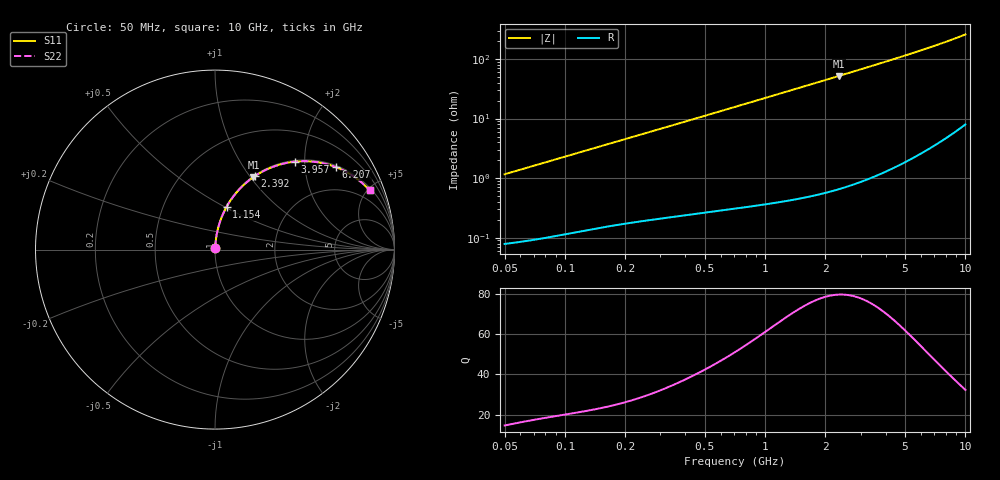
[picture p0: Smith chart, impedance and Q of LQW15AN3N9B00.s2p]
!Murata Part Number: LQW15AN3N9B00
!These Parameters are Measured in Series Mode Connection
!  o--[Z]--o
!Port1  Port2
!  o-------o
!Freq. Start=50[MHz] Stop=10[GHz], 401[Steps]
# Hz S RI R 50
!Freq.(Hz)	S 11(Real)	S 11(Imag)	S 21(Real)	S 21(Imag)	S 12(Real)	S 12(Imag)	S 22(Real)	S 22(Imag)
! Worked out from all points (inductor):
!   401 points, 50 MHz to 10 GHz, reference 50 ohm
!   read as one part in series: L = 3.68 nH near 51.34 MHz
!   highest Q = 79.5 at 2.329 GHz (marker M1), where L = 3.54 nH
!   S11 on the Smith chart (normalised r, x): 50 MHz: 1.00, +0.02; 1.154 GHz: 1.01, +0.51; 2.392 GHz: 1.01, +1.06; 3.957 GHz: 1.03, +1.78; 6.207 GHz: 1.06, +2.90; 10 GHz: 1.16, +5.16
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5e7  0.000921 0.0116  0.9991 -0.0116  0.9991 -0.0116  0.000921 0.0116
1.214486e8  0.00205 0.0276  0.9979 -0.0276  0.9979 -0.0276  0.00205 0.0276
1.956524e8  0.00364 0.0439  0.9964 -0.0439  0.9964 -0.0439  0.00364 0.0439
2.949953e8  0.00639 0.0655  0.9936 -0.0655  0.9936 -0.0655  0.00639 0.0655
4.689809e8  0.0132 0.1028  0.9868 -0.1028  0.9868 -0.1028  0.0132 0.1028
7.071068e8  0.0269 0.1522  0.9731 -0.1522  0.9731 -0.1522  0.0269 0.1522
9.215873e8  0.0431 0.1947  0.9569 -0.1947  0.9569 -0.1947  0.0431 0.1947
1.154331e9  0.0645 0.2381  0.9355 -0.2381  0.9355 -0.2381  0.0645 0.2381
1.426828e9  0.094 0.2849  0.906 -0.2849  0.906 -0.2849  0.094 0.2849
1.717543e9  0.1297 0.3295  0.8703 -0.3295  0.8703 -0.3295  0.1297 0.3295
2.013439e9  0.1694 0.3688  0.8306 -0.3688  0.8306 -0.3688  0.1694 0.3688
2.329253e9  0.2142 0.404  0.7858 -0.404  0.7858 -0.404  0.2142 0.404
2.391784e9  0.2232 0.4102  0.7768 -0.4102  0.7768 -0.4102  0.2232 0.4102
2.730534e9  0.2727 0.4391  0.7273 -0.4391  0.7273 -0.4391  0.2727 0.4391
3.158828e9  0.3349 0.4655  0.6651 -0.4655  0.6651 -0.4655  0.3349 0.4655
3.956578e9  0.4439 0.4898  0.5561 -0.4898  0.5561 -0.4898  0.4439 0.4898
4.171863e9  0.4711 0.4919  0.5289 -0.4919  0.5289 -0.4919  0.4711 0.4919
5.088839e9  0.5746 0.4863  0.4254 -0.4863  0.4254 -0.4863  0.5746 0.4863
6.207365e9  0.6742 0.4592  0.3258 -0.4592  0.3258 -0.4592  0.6742 0.4592
7.983737e9  0.7844 0.3994  0.2156 -0.3994  0.2156 -0.3994  0.7844 0.3994
9.114482e9  0.8325 0.3598  0.1675 -0.3598  0.1675 -0.3598  0.8325 0.3598
1e10  0.8618 0.33  0.1382 -0.33  0.1382 -0.33  0.8618 0.33
